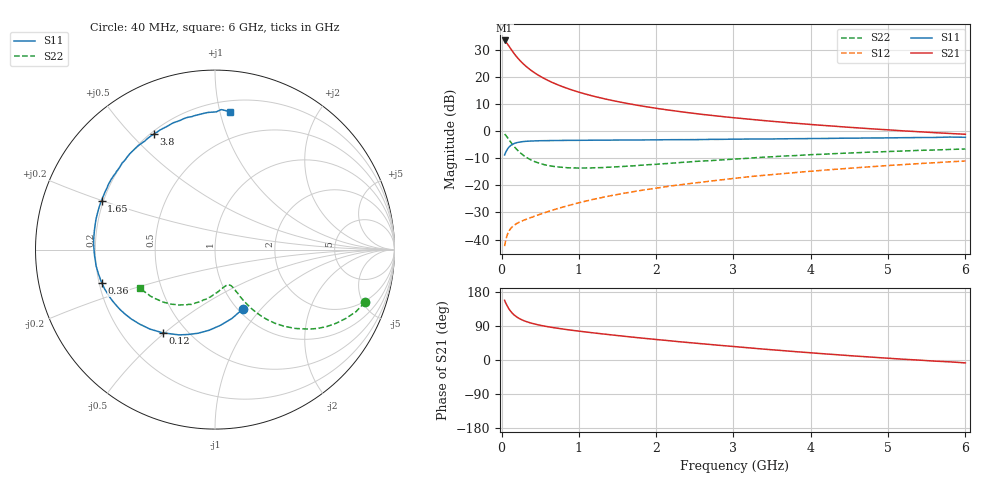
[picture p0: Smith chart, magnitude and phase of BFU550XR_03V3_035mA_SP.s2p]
! Filename:  P:\Prog\Test\Noise\ATS_data\Testdata_Net\03 Spar\BFU550XR_APG2013_45_C05_03p3V_035mA_SP_CM01_D.s2p
! Date/Time: Tue 06/Aug/2013 14:38:15
! BFU550XR_APG2013_45_C05_03p3V_25to35mA_SP_CM01_Bias2_R.s2p
! MDIF S-parameter v. bias file
! BFU550XR_APG2013_45_C05_03p3V_25to35mA_SP_CM01
! Date/time Mon Aug 05 16:35:29 2013
! VAR V_out= 3.3000
! VAR I_out= 34.9950
! VAR V_in= 0.8501
! VAR I_in= 0.4129
! Device data file deembeded for feedlines and parallel
! Original file: \03 Spar\BFU550XR_APG2013_45_C05_03p3V_035mA_SP_CM01_R.s2p
! Feed-files: PR006V01_02082013_Feed1.s2p, PR006V01_02082013_Feed2.s2p
! Parallel-file: PR006V01_02082013_Par.s2p
# MHz S MA R 50
!  Freq-MHz  S11-mag  S11-arg  S21-mag  S21-arg  S12-mag  S12-arg  S22-mag  S22-arg
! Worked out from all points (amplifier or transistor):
!   98 points, 40 MHz to 6 GHz, reference 50 ohm
!   highest |S21| = 33.5 dB at 40 MHz (marker M1)
!   |S21| within 3 dB of that: start of sweep to 117.5 MHz
!   unconditionally stable (mu >= 1): 830 MHz to 2.876 GHz
!   at 300 MHz: K = 0.64, MSG = 28.6 dB, |S12| = -32.7 dB
!   at 1.6 GHz: K = 1.06, MAG = 15.1 dB, |S12| = -22.8 dB
!   at 6 GHz: K = 0.80, MSG = 4.9 dB, |S12| = -11.0 dB
!   S11 on the Smith chart (normalised r, x): 40 MHz: 1.05, -0.80; 120 MHz: 0.37, -0.49; 360 MHz: 0.21, -0.14; 1.65 GHz: 0.19, +0.20; 3.8 GHz: 0.21, +0.58; 6 GHz: 0.28, +1.07
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40  0.3656 -65.1  47.55 157.6  0.007536 72.9  0.8854 -19.4
50  0.3953 -76.3  45.65 152.2  0.009105 69.6  0.8581 -23.8
70  0.4506 -94.2  42.13 144.2  0.01168 63.4  0.7893 -31.4
80  0.4754 -101.4  40.26 140.3  0.0128 61.0  0.7554 -34.6
100  0.5158 -112.9  36.59 133.7  0.01459 56.8  0.6878 -40.1
120  0.5477 -122.2  33.26 128.1  0.01602 53.8  0.6271 -44.5
140  0.5725 -129.3  30.28 123.4  0.01721 51.7  0.5745 -48.0
160  0.5903 -135.3  27.59 119.5  0.01821 50.2  0.5302 -50.8
180  0.6053 -140.2  25.34 116.1  0.01908 49.3  0.4905 -53.1
220  0.626 -147.9  21.7 110.6  0.02053 48.4  0.4279 -56.3
280  0.6444 -156.1  17.68 104.5  0.02247 48.7  0.362 -59.3
360  0.6576 -163.6  14.11 98.8  0.02485 50.5  0.3064 -61.5
480  0.667 -171.1  10.77 92.6  0.02871 53.7  0.2592 -63.4
650  0.673 -178.5  8.042 86.1  0.03447 57.8  0.2271 -65.2
1050  0.6809 169.8  5.029 74.9  0.04968 63.1  0.2094 -71.1
1650  0.6886 156.6  3.218 61.3  0.07423 64.8  0.2278 -82.9
2050  0.6959 148.9  2.591 53.2  0.09107 64.4  0.2493 -90.6
3100  0.7158 129.8  1.725 33.8  0.1393 60.0  0.311 -108.7
3800  0.7285 117.8  1.405 22.1  0.1726 55.0  0.355 -120.0
4100  0.7349 112.9  1.3 17.4  0.1874 52.7  0.3735 -124.5
5200  0.7602 95.4  1.016 2.0  0.2423 43.4  0.432 -141.0
6000  0.7732 83.9  0.8791 -7.6  0.2822 35.6  0.4702 -153.0
